(* Logix 5000 Rung export; software revision 16.03 *)

TYPE MCMRClockType :   // Allows read/write of clock value between the module and processor
STRUCT
   Read : BOOL;   // Reads current time from the module
   Write : BOOL;   // Writes current time from the module
   Config : MCMRDateTime;   // Date and time configuration read or written between the module and processor
END_STRUCT
END_TYPE

TYPE MCMREthernet :   // Stores the MVI56E-MCMR IP settings
STRUCT
   IP : INT[4];
   Netmask : INT[4];
   Gateway : INT[4];
END_STRUCT
END_TYPE

TYPE MCMRDateTime :   // Stores the date and time value
STRUCT
   Year : DINT;
   Month : DINT;
   Day : DINT;
   Hour : DINT;
   Minute : DINT;
   Seconds : DINT;
END_STRUCT
END_TYPE

TYPE MCMREthernetType :   // Allows read/write Ethernet settings between the module and processor
STRUCT
   Read : BOOL;   // Enable Ethernet configuration transfer from module to processor
   Write : BOOL;   // Enable Ethernet configuration transfer from processor to module
   Config : MCMREthernet;
END_STRUCT
END_TYPE

ADD_ON_INSTRUCTION AOI56EMCMR_Optional   (* revision 1.2, vendor ProSoft Technology Inc. *)
// MVI56E-MCMR Optional Add-On Ethernet/Clock.
// Revision note:
// v1.2 - Updated name and description for standardization. No feature changes.
VAR_IN_OUT
   MVI56MCMREthernet : MCMREthernetType; {required}   // MVI56E-MCM Rev2 Ethernet Settings
   MVI56MCMRClock : MCMRClockType; {required}   // MVI56E-MCM Rev2 Clock Settings
   ReadEthernetMSG : MESSAGE; {required}   // Read Ethernet Settings Message
   WriteEthernetMSG : MESSAGE; {required}   // Write Ethernet Settings Message
   ReadClockMSG : MESSAGE; {required}   // Read Clock Settings Message
   WriteClockMSG : MESSAGE; {required}   // Write Clock Settings Message
END_VAR

ROUTINE Logic   (* ladder *)
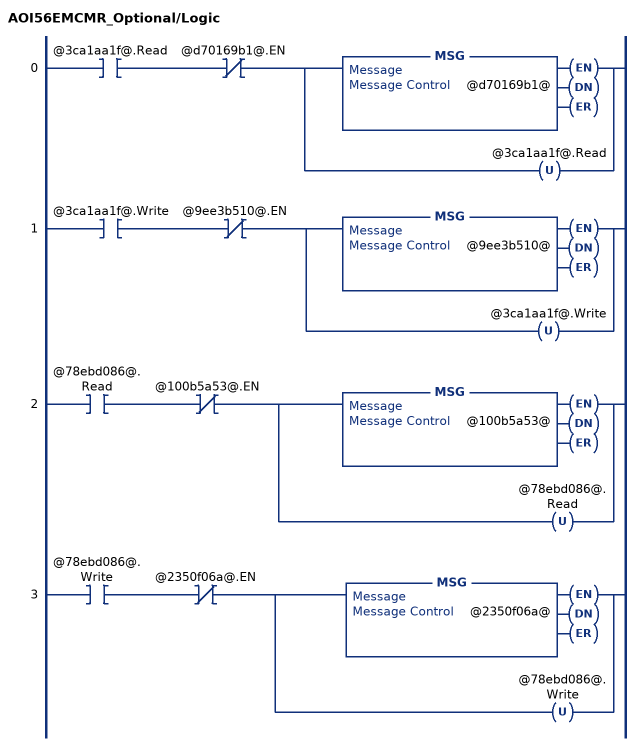
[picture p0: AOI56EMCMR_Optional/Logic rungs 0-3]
   0: XIC(@3ca1aa1f@.Read)XIO(@d70169b1@.EN)[MSG(@d70169b1@) ,OTU(@3ca1aa1f@.Read) ];
   1: XIC(@3ca1aa1f@.Write)XIO(@9ee3b510@.EN)[MSG(@9ee3b510@) ,OTU(@3ca1aa1f@.Write) ];
   2: XIC(@78ebd086@.Read)XIO(@100b5a53@.EN)[MSG(@100b5a53@) ,OTU(@78ebd086@.Read) ];
   3: XIC(@78ebd086@.Write)XIO(@2350f06a@.EN)[MSG(@2350f06a@) ,OTU(@78ebd086@.Write) ];
END_ROUTINE
END_ADD_ON_INSTRUCTION

VAR_GLOBAL   (* controller tags *)
   ReadClockMSG : MESSAGE;
        MessageParameters(MessageType := CIP Generic, ConnectedFlag := 2, ConnectionPath := MCMR, ServiceCode := 16#000e, ObjectType := 16#0004, TargetObject := 8, AttributeNumber := 16#0020, DestinationTag := MVI56EMCMRClock.Config)
   AOI56EMCMR_Optional : AOI56EMCMR_Optional;
   MVI56EMCMRClock : MCMRClockType;
   WriteClockMSG : MESSAGE;
        MessageParameters(MessageType := CIP Generic, RequestedLength := 24, ConnectedFlag := 2, ConnectionPath := MCMR, ServiceCode := 16#0010, ObjectType := 16#0004, TargetObject := 8, AttributeNumber := 16#0020, LocalElement := MVI56EMCMRClock.Config)
   MVI56EMCMREthernet : MCMREthernetType;
   ReadEthernetMSG : MESSAGE;
        MessageParameters(MessageType := CIP Generic, ConnectedFlag := 2, ConnectionPath := MCMR, ServiceCode := 16#000e, ObjectType := 16#0004, TargetObject := 8, DestinationTag := MVI56EMCMREthernet.Config)
   WriteEthernetMSG : MESSAGE;
        MessageParameters(MessageType := CIP Generic, RequestedLength := 24, ConnectedFlag := 2, ConnectionPath := MCMR, ServiceCode := 16#0010, ObjectType := 16#0004, TargetObject := 8, LocalElement := MVI56EMCMREthernet.Config)
END_VAR

PROGRAM MainProgram

ROUTINE MainRoutine   (* ladder *)
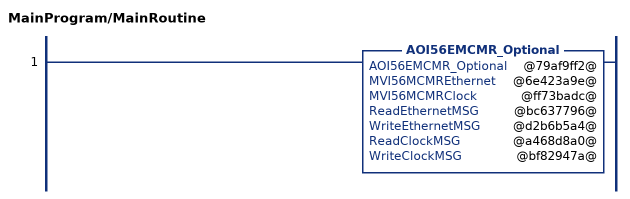
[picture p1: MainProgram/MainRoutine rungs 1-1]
   1: AOI56EMCMR_Optional(@79af9ff2@,@6e423a9e@,@ff73badc@,@bc637796@,@d2b6b5a4@,@a468d8a0@,@bf82947a@);
END_ROUTINE
END_PROGRAM
